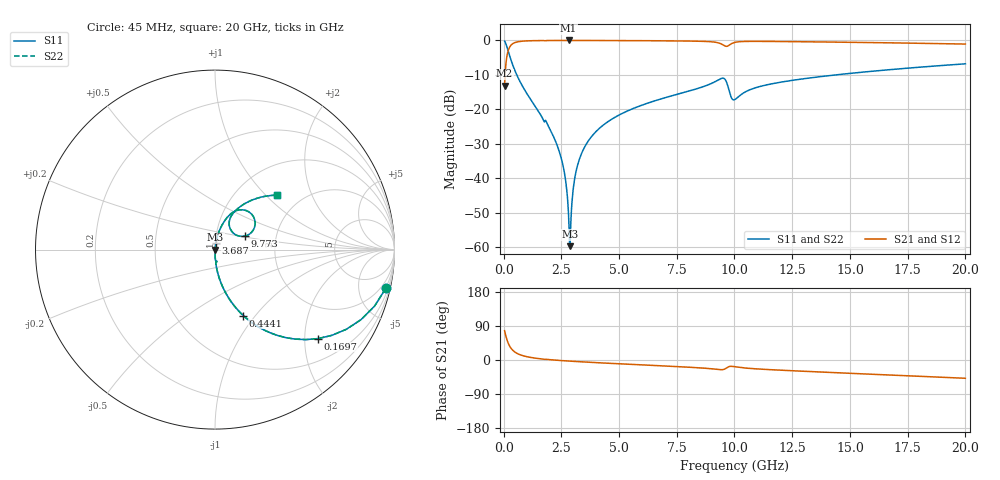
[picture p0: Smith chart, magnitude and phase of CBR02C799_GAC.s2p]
! S-parameter model data by Modelithics Inc.  support@modelithics.com 813-866-6335  Tampa FL USA
! S-Parameter data specifications:
! Substrate: 20-mil Rogers 4350B, substrate thickness, H=0.508mm, Dielectric constant, Er=3.75
! PCB Mounting Pad Footprint: Pad width, PadW=0.32mm , Pad length, PadL=0.37mm , Pad gap, PadG (edge-to-edge)=0.19mm , Reference planes=0.93mm apart
#  GHz  S  MA  R 50
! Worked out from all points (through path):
!   801 points, 45 MHz to 20 GHz, reference 50 ohm
!   highest |S21| = -0.01 dB at 2.814 GHz (marker M1); lowest = -13.1 dB at 45 MHz (marker M2)
!   group delay of S21, straight-line fit = 8.26 ps
!   lowest |S11| = -59.7 dB at 2.864 GHz (marker M3), VSWR 1.00, Z = 50.1 - j0.0392 ohm
!   |S11| at or under -10 dB: 571.9 MHz to 14.38 GHz (13.81 GHz wide, 185 % of centre)
!   |S22| runs from -59.7 to -0.2 dB; largest |S21 - S12| = 0
!   S11 on the Smith chart (normalised r, x): 45 MHz: 0.99, -8.80; 169.7 MHz: 0.99, -2.32; 444.1 MHz: 0.99, -0.87; 3.687 GHz: 1.01, +0.07; 9.773 GHz: 1.38, +0.22; 20 GHz: 1.51, +1.16
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0.045  0.9753 -12.8  0.221 77.2  0.221 77.2  0.9753 -12.8
0.169719  0.759 -40.8  0.6507 49.2  0.6507 49.2  0.759 -40.8
0.294438  0.555 -56.5  0.8313 33.4  0.8313 33.4  0.555 -56.5
0.4441  0.3999 -66.8  0.916 23.1  0.916 23.1  0.3999 -66.8
1.092637  0.1533 -82.0  0.9874 7.7  0.9874 7.7  0.1533 -82.0
2.314881  0.03046 -88.9  0.9986 -0.7  0.9986 -0.7  0.03046 -88.9
2.63915  0.01184 -87.4  0.9989 -2.1  0.9989 -2.1  0.01184 -87.4
2.813756  0.002972 -73.6  0.999 -2.8  0.999 -2.8  0.002972 -73.6
2.863644  0.001041 -22.1  0.999 -3.0  0.999 -3.0  0.001041 -22.1
2.938475  0.003426 69.9  0.9989 -3.3  0.9989 -3.3  0.003426 69.9
3.113081  0.01144 81.0  0.9989 -3.9  0.9989 -3.9  0.01144 81.0
3.387462  0.02339 82.6  0.9986 -4.9  0.9986 -4.9  0.02339 82.6
3.686787  0.03559 82.4  0.9982 -5.9  0.9982 -5.9  0.03559 82.4
4.784313  0.07554 79.8  0.9959 -9.3  0.9959 -9.3  0.07554 79.8
6.704981  0.1382 74.4  0.9886 -15.0  0.9886 -15.0  0.1382 74.4
9.448794  0.2824 48.0  0.8825 -25.6  0.8825 -25.6  0.2824 48.0
9.773062  0.1839 24.2  0.8544 -17.2  0.8544 -17.2  0.1839 24.2
10.0225  0.1392 49.4  0.9378 -17.8  0.9378 -17.8  0.1392 49.4
11.04519  0.2123 64.1  0.9691 -23.8  0.9691 -23.8  0.2123 64.1
13.36496  0.2887 58.6  0.9539 -30.7  0.9539 -30.7  0.2887 58.6
16.68248  0.3759 50.0  0.9236 -39.5  0.9236 -39.5  0.3759 50.0
20  0.4581 41.4  0.8857 -48.2  0.8857 -48.2  0.4581 41.4
